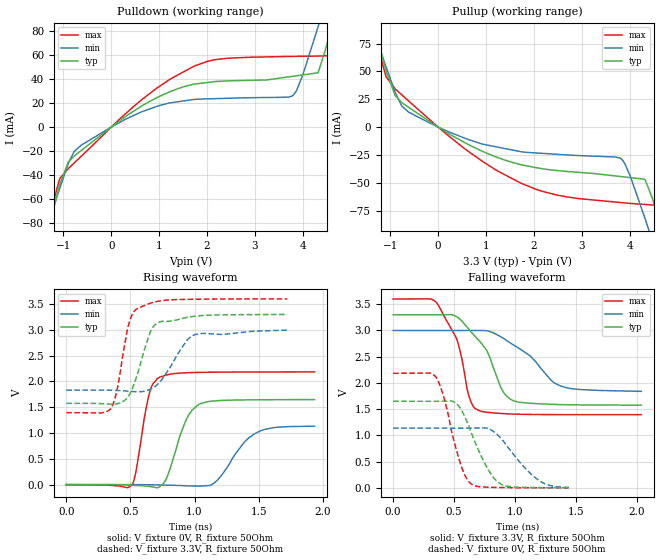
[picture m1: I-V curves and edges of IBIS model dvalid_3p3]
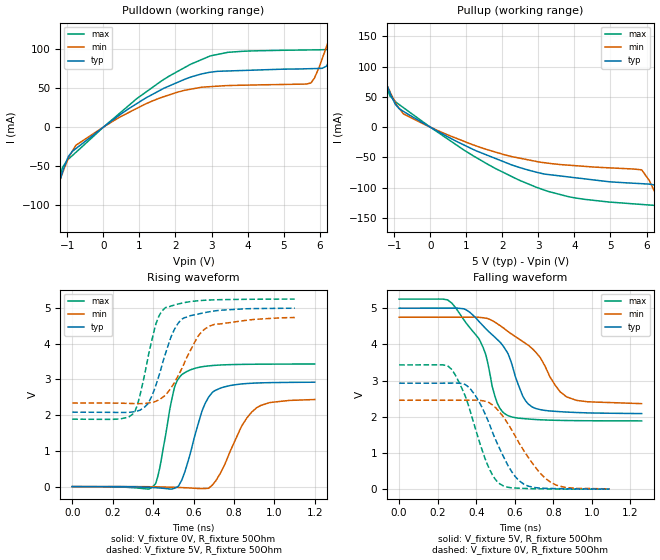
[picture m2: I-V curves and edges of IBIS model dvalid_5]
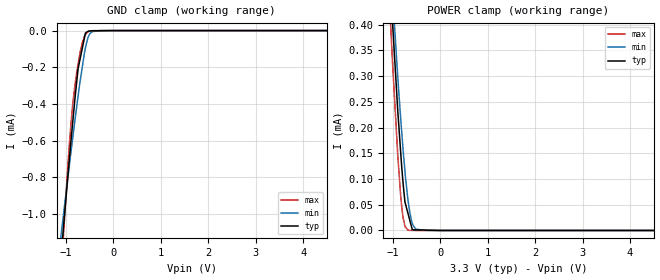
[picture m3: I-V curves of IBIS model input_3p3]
|Texas Instruments Incorporated
| DDC114: Quad Current Input 20-Bit Analog-To-Digital Converter
| Marketing part#   Digital Voltage Range   Package-type   #pins
| DDC114IRTCR   2.7V-5.25V   VQFN   48
| DDC114IRTCRG3   2.7V-5.25V   VQFN   48
| DDC114IRTCT   2.7V-5.25V   VQFN   48
| DDC114IRTCTG3   2.7V-5.25V   VQFN   48
[IBIS Ver]   3.2
[File name]   ddc114.ibs
|SIMDE Ver   V3.0 - 201101 - RHL4 - Build 457
[File Rev]   1.0
[Date]   7/13/2011
[Source]
| Texas Instruments Incorporated.
| Analog-eLab Design Center, HPA
| 12500 TI Blvd
| Dallas, TX -75243
| e-mail: elab_scm_ibis@list.ti.com
[Notes]   Revision History:
| Rev 1.0: 7/13/2011
| - Initial version of the model
| - Model generated from simulations in TISPICE
| - Model matched to SPICE simulation
| - C_comp although listed in numerical order of value are
|   obtained from varying PVT conditions. For PVT conditions for
|   each specific value refer the buffer description under
|   respective [Model]. IBIS model user is responsible for using
|   appropriate C_comp to simulate for Signal Integrity.
| - Model names with a trailing _3p3 contains the model for
|   3.3V [3.0V and 3.6V]. Model names with a trailing _5 contains
|   the model for 5.0V [4.75V and 5.25V].
|*  EXCEPTION:   *
|*  - For model RESET there will be a leakage current in the   *
|*   clamp I-V table because of the pullup on pad.   *
[Disclaimer]
| This model is designed as an aid for customers of Texas Instruments.
| TI and its licensors and suppliers make no warranties, either expressed
| or implied, with respect to this  model, including the warranties of
| merchantability or fitness for a particular purpose. The model is
| provided solely on an "as is" basis. The entire risk as to its quality
| and performance is with the customer.
[Copyright]
 (C) Copyright 2011 Texas Instruments Incorporated.All rights reserved.
|   DDC114
[Component]   DDC114
[Manufacturer]   TI
[Package]   |48 VQFN  -  RTC package
|   typ   min   max
R_pkg   0.07335   0.06625   0.09331
L_pkg   1.25878nH   1.11691nH   1.65971nH
C_pkg   0.40216pF   0.37695pF   0.45725pF
[Pin]  signal_name   model_name   R_pin   L_pin   C_pin
1   DOUT   DOUT_DVALID   0.07718   1.33291nH  0.43988pF
2   _DOUT   DOUT_DVALID   0.07236   1.23651nH  0.40395pF
3   CLK_4X   INPUT   0.06871   1.16431nH  0.40738pF
4   FORMAT   INPUT   0.06661   1.12331nH  0.39420pF
5   HISPD/_LOPWR   INPUT   0.06625   1.11691nH  0.38235pF
6   RANGE0   INPUT   0.06711   1.13471nH  0.37695pF
7   RANGE1   INPUT   0.06859   1.16501nH  0.37885pF
8   RANGE2   INPUT   0.07053   1.20411nH  0.38749pF
9   AGND   GND   0.07256   1.24541nH  0.40171pF
10   VREF   TERM   0.07469   1.28841nH  0.41402pF
11   AGND   GND   0.07881   1.37201nH  0.41890pF
12   AGND   GND   0.09121   1.62491nH  0.46203pF
13   AGND   GND   0.08470   1.49191nH  0.45195pF
14   AGND   GND   0.07477   1.29131nH  0.41332pF
15   AIN4   TERM   0.07121   1.22011nH  0.40949pF
16   AGND   GND   0.07069   1.20981nH  0.40042pF
17   AIN3   TERM   0.06914   1.17901nH  0.38622pF
18   AGND   GND   0.06992   1.19441nH  0.38292pF
19   AGND   GND   0.07038   1.20361nH  0.39011pF
20   AGND   GND   0.07481   1.29231nH  0.39558pF
21   AIN2   TERM   0.07296   1.25531nH  0.40408pF
22   AGND   GND   0.07964   1.38951nH  0.42187pF
23   AIN1   TERM   0.08099   1.41681nH  0.41365pF
24   AGND   GND   0.08669   1.53211nH  0.44910pF
25   AGND   GND   0.08782   1.55561nH  0.45732pF
26   AGND   GND   0.07613   1.31761nH  0.41270pF
27   AVDD   POWER   0.07504   1.29551nH  0.41279pF
28   AGND   GND   0.07369   1.26821nH  0.40112pF
29   DGND   GND   0.07069   1.20751nH  0.38902pF
30   DGND   GND   0.06871   1.16731nH  0.37769pF
31   TEST   INPUT   0.06717   1.13591nH  0.37772pF
32   _RESET   RESET   0.06625   1.11691nH  0.37891pF
33   NC   NC   0.00005   0.00141nH  0.31967pF
34   NC   NC   0.00005   0.00141nH  0.32949pF
35   _DIN   DIN   0.08700   1.53131nH  0.41889pF
36   DIN   DIN   0.09331   1.65971nH  0.45725pF
37   DVDD   POWER   0.08459   1.48251nH  0.44764pF
38   DGND   GND   0.04204   1.02189nH  0.46866pF
39   _DCLK   INPUT   0.08351   1.46051nH  0.42645pF
40   DCLK   INPUT   0.07808   1.35021nH  0.41213pF
41   DGND   GND   0.07472   1.28211nH  0.39060pF
42   CLK   CLK   0.07247   1.23681nH  0.38444pF
43   DGND   GND   0.07058   1.19861nH  0.38161pF
44   _DVALID   DOUT_DVALID   0.06925   1.17211nH  0.38411pF
45   DGND   GND   0.06900   1.16711nH  0.39824pF
46   CONV   INPUT   0.07026   1.19231nH  0.40906pF
47   DGND   GND   0.07318   1.25121nH  0.40470pF
48   DGND   GND   0.07736   1.33561nH  0.43945pF
49   THERMAL_PAD   NC   0.00005   0.00141nH  6.11239pF
[Diff_pin]   inv_pin   vdiff   tdelay_typ   tdelay_min   tdelay_max
1   2   NA   NA   NA   NA
36   35   NA   NA   NA   NA
40   39   NA   NA   NA   NA
|   Model Selectors
[Model Selector] DOUT_DVALID
dvalid_3p3   3.3V digital output
dvalid_5   5.0V digital output
[Model Selector] INPUT
input_3p3   3.3V digital input
input_5   5.0V digital input
[Model Selector] RESET
reset_3p3   3.3V digital input
reset_5   5.0V digital input
[Model Selector] DIN
din_3p3   3.3V digital input
din_5   5.0V digital input
[Model Selector] CLK
clk_3p3   3.3V digital input
clk_5   5.0V digital input
[Model Selector] TERM
term_3-3V   3.3V nominal termination
term_5-0V   5.0V nominal termination
[Model] term_3-3V
Model_type Terminator
C_comp   1.0e-20F  1.0e-20F  1.0e-20F
|   typ   min   max
[Voltage Range]   3.3V   3.0V   3.6V
[POWER Clamp Reference]   3.3V   3.0V   3.6V
[GND Clamp Reference]   0V   0V   0V
|Ambient Temperature   25   85   -40
|Junction Temperature
[Temperature Range]   27   87   -40
[Model] term_5-0V
Model_type Terminator
C_comp   1.0e-20F  1.0e-20F  1.0e-20F
|   typ   min   max
[Voltage Range]   5.0V   4.75V   5.25V
[POWER Clamp Reference]   5.0V   4.75V   5.25V
[GND Clamp Reference]   0V   0V   0V
|Ambient Temperature   25   85   -40
|Junction Temperature
[Temperature Range]   27   87   -40
| Models and submodels in the file (12): dvalid_3p3 (Output), dvalid_5 (Output), input_3p3 (Input), input_5 (Input), reset_3p3 (Input), reset_5 (Input), din_3p3 (Input), din_5 (Input), clk_3p3 (Input), clk_5 (Input), term_3-3V (Terminator), term_5-0V (Terminator)
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|   dvalid_3p3 Model
[Model]   dvalid_3p3
Model_type   Output
Polarity   Non-Inverting
Vmeas = 1.65
Vref = 1.65
Cref = 9pF
Rref = 50
|   typ   min   max
|   (nom PVT)   (fast PVT)   (slow PVT)
|C_comp from frequency sweep method (F=8MHz)
|C_comp   8.990e-13   8.643e-13   9.187e-13
|ON state : BUFFER OUTPUT TURNED HIGH
|C_comp   8.990e-13   8.643e-13   9.187e-13
|OFF state: BUFFER OUTPUT TURNED LOW
|C_comp   8.386e-13   7.914e-13   9.617e-13
|C_comp from LC tank measurement(L=1nH)
|Resonant Frequency(Hz)   9.340e+09   9.530e+09   9.090e+09
C_comp   2.907e-13   2.792e-13   3.069e-13
|ON state : BUFFER OUTPUT TURNED HIGH
|Resonant Frequency(Hz)   9.340e+09   9.530e+09   9.090e+09
|C_comp   2.907e-13   2.792e-13   3.069e-13
|OFF state: BUFFER OUTPUT TURNED LOW
|Resonant Frequency(Hz)   9.920e+09   9.990e+09   9.480e+09
|C_comp   2.577e-13   2.541e-13   2.821e-13
| Where nom  PVT is Nominal Process, 3.3V, 27C
|   Fast PVT is Strong Process,  3.6V, -40C
|   Slow PVT is Weak Process,   3V, 87C
[Voltage Range]   3.3   3   3.6
|Ambient Temperature   25   85   -40
|Junction Temperature
[Temperature Range]   27   87   -40
[Pullup Reference]   3.3   3   3.6
[Pulldown Reference]   0   0   0
[Power Clamp Reference]   3.3   3   3.6
[GND Clamp Reference]   0   0   0
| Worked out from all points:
|   slope of the pulldown table from 0 to 0.495 V, typ, clamps not added: 35.3 ohm
|   slope of the pullup table from 0 to 0.495 V, typ, clamps not added: 39.5 ohm
|   falling waveform, V_fixture 3.3V, R_fixture 50Ohm: 20-80 % time 235ps typ, 331ps min, 167ps max; typ from 3.3 V to 1.58 V
|   rising waveform, V_fixture 0V, R_fixture 50Ohm: 20-80 % time 135ps typ, 199ps min, 89.7ps max; typ from 0 V to 1.65 V
|   rising waveform, V_fixture 3.3V, R_fixture 50Ohm: 20-80 % time 130ps typ, 177ps min, 96.6ps max; typ from 1.58 V to 3.3 V
|   falling waveform, V_fixture 0V, R_fixture 50Ohm: 20-80 % time 190ps typ, 249ps min, 143ps max; typ from 1.65 V to 0.002 V
[Pulldown]
|   Voltage   I(typ)   I(min)   I(max)
-3.3V     -409.1mA   -351.2mA   -450.8mA
-1.409V   -98.56mA   -93.91mA   -95.86mA
-1.307V   -82.51mA   -80.61mA   -77.63mA
-1.069V   -47.29mA   -50.4mA    -42.8mA
-636mV    -19.86mA   -15.41mA   -24.74mA
1.75V     36.04mA    23.17mA    51.28mA
3.78V     42.43mA    26.05mA    59.14mA
4.316V    45.43mA    83.87mA    59.41mA
4.748V    107.6mA    142mA      61.58mA
4.9V      132.2mA    162.7mA    80.33mA
5.168V    175.9mA    199.9mA    128.8mA
6.6V      415mA      398.6mA    399.1mA
[Pullup]
|   Voltage   I(typ)   I(min)   I(max)
-3.3V     414.9mA    356.7mA    456.5mA
-1.435V   104.9mA    99.57mA    103.2mA
-1.087V   50.96mA    53.97mA    45.12mA
-897.6mV  28.24mA    31.11mA    34.26mA
-624mV    17.96mA    13.67mA    23.73mA
1.746V    -34.06mA   -22.28mA   -50.75mA
3.804V    -44.43mA   -27.97mA   -67.79mA
4.316V    -46.91mA   -81.93mA   -69.55mA
4.468V    -63.59mA   -101.9mA   -70mA
4.81V     -115.6mA   -147.6mA   -73.38mA
4.954V    -138.3mA   -167mA     -89.55mA
6.6V      -409.3mA   -392.5mA   -394.1mA
[Ramp]
R_load = 50
|   typ   min   max
dV/dt_r   0.990295/1.3557e-10   0.68271/2.0008e-10   1.31056/8.9629e-11
dV/dt_f   1.0346/2.35346e-10   0.700849/3.32929e-10   1.32291/1.66806e-10
[Falling Waveform]
V_fixture = 3.3V
V_fixture_min = 3V
V_fixture_max = 3.6V
R_fixture = 50Ohm
|   Time   V(typ)   V(min)   V(max)
0s        3.3V       3V         3.6V
358ps     3.3V       3V         3.525V
520ps     3.264V     3V         2.851V
622ps     3.025V     3.001V     1.754V
710ps     2.797V     3V         1.47V
778ps     2.573V     2.991V     1.439V
892ps     1.88V      2.869V     1.417V
986ps     1.664V     2.728V     1.407V
1.37ns    1.588V     1.947V     1.397V
2.038ns   1.577V     1.84V      1.395V
[Rising Waveform]
V_fixture = 0V
V_fixture_min = 0V
V_fixture_max = 0V
R_fixture = 50Ohm
|   Time   V(typ)   V(min)   V(max)
0s        1.108nV    1.352nV    1.021nV
510ps     -11.02mV   559.2uV    -5.106mV
648ps     -35.21mV   -2.127mV   1.774V
726ps     -43.97mV   -6.168mV   2.081V
790ps     174.6mV    -10.63mV   2.13V
940ps     1.285V     -23.37mV   2.168V
1.032ns   1.552V     -27.83mV   2.175V
1.176ns   1.627V     83.58mV    2.179V
1.46ns    1.643V     974.4mV    2.183V
1.934ns   1.648V     1.132V     2.184V
[Rising Waveform]
V_fixture = 3.3V
V_fixture_min = 3V
V_fixture_max = 3.6V
R_fixture = 50Ohm
|   Time   V(typ)   V(min)   V(max)
0s        1.576V     1.831V     1.395V
350ps     1.56V      1.829V     1.477V
398ps     1.568V     1.824V     1.859V
480ps     1.693V     1.811V     3.044V
550ps     2.104V     1.801V     3.406V
654ps     2.954V     1.846V     3.515V
720ps     3.143V     1.964V     3.556V
938ps     3.24V      2.788V     3.59V
996ps     3.262V     2.901V     3.592V
1.722ns   3.297V     2.993V     3.6V
[Falling Waveform]
V_fixture = 0V
V_fixture_min = 0V
V_fixture_max = 0V
R_fixture = 50Ohm
|   Time   V(typ)   V(min)   V(max)
0s        1.651V     1.139V     2.184V
350ps     1.65V      1.139V     2.12V
424ps     1.652V     1.138V     1.666V
520ps     1.603V     1.138V     720mV
582ps     1.39V      1.138V     279.8mV
640ps     1.066V     1.14V      77.63mV
774ps     375.5mV    1.137V     14.08mV
888ps     67.93mV    939.3mV    6.722mV
1.21ns    5.107mV    120.8mV    1.565mV
1.442ns   2.095mV    8.586mV    925.5uV
|   dvalid_5 Model
[Model]   dvalid_5
Model_type   Output
Polarity   Non-Inverting
Vmeas = 2.5
Vref = 2.5
Cref = 9pF
Rref = 50
|   typ   min   max
|   (nom PVT)   (fast PVT)   (slow PVT)
|C_comp from frequency sweep method (F=8MHz)
|C_comp   8.665e-13   7.977e-13   9.259e-13
|ON state : BUFFER OUTPUT TURNED HIGH
|C_comp   8.665e-13   7.977e-13   9.259e-13
|OFF state: BUFFER OUTPUT TURNED LOW
|C_comp   7.892e-13   7.024e-13   8.409e-13
|C_comp from LC tank measurement(L=1nH)
|Resonant Frequency(Hz)   9.120e+09   9.140e+09   9.060e+09
C_comp   3.048e-13   3.035e-13   3.089e-13
|ON state : BUFFER OUTPUT TURNED HIGH
|Resonant Frequency(Hz)   9.120e+09   9.140e+09   9.060e+09
|C_comp   3.048e-13   3.035e-13   3.089e-13
|OFF state: BUFFER OUTPUT TURNED LOW
|Resonant Frequency(Hz)   1.011e+10   1.026e+10   9.970e+09
|C_comp   2.481e-13   2.409e-13   2.551e-13
| Where nom  PVT is Nominal Process, 5V, 27C
|   Fast PVT is Strong Process,  5.25V, -40C
|   Slow PVT is Weak Process,   4.75V, 87C
[Voltage Range]   5   4.75   5.25
|Ambient Temperature   25   85   -40
|Junction Temperature
[Temperature Range]   27   87   -40
[Pullup Reference]   5   4.75   5.25
[Pulldown Reference]   0   0   0
[Power Clamp Reference]   5   4.75   5.25
[GND Clamp Reference]   0   0   0
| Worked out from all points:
|   slope of the pulldown table from 0 to 0.75 V, typ, clamps not added: 29.9 ohm
|   slope of the pullup table from 0 to 0.75 V, typ, clamps not added: 31.1 ohm
|   falling waveform, V_fixture 5V, R_fixture 50Ohm: 20-80 % time 182ps typ, 227ps min, 148ps max; typ from 5 V to 2.09 V
|   rising waveform, V_fixture 0V, R_fixture 50Ohm: 20-80 % time 92.2ps typ, 125ps min, 66.2ps max; typ from 0 V to 2.92 V
|   rising waveform, V_fixture 5V, R_fixture 50Ohm: 20-80 % time 104ps typ, 134ps min, 80.1ps max; typ from 2.08 V to 4.99 V
|   falling waveform, V_fixture 0V, R_fixture 50Ohm: 20-80 % time 150ps typ, 178ps min, 129ps max; typ from 2.93 V to 0.004 V
[Pulldown]
|   Voltage   I(typ)   I(min)   I(max)
-5V       -692.7mA   -587mA     -774.9mA
-2.336V   -249.9mA   -219.4mA   -268.2mA
-1.31V    -83.5mA    -81.13mA   -78.77mA
-1.129V   -56.99mA   -58.26mA   -51.14mA
-760mV    -27.41mA   -23.18mA   -32.26mA
1.149V    36.72mA    29.39mA    44.02mA
2.94V     70.4mA     51.94mA    90.99mA
5.752V    75.1mA     56.65mA    99.19mA
6.195V    78.52mA    104.1mA    99.67mA
6.525V    122.3mA    147.1mA    100.7mA
7.088V    213.8mA    225mA      179.3mA
10V       701.9mA    630.5mA    736.1mA
[Pullup]
|   Voltage   I(typ)   I(min)   I(max)
-5V       701.6mA    595.7mA    784.1mA
-2.336V   253.8mA    223.3mA    272mA
-1.31V    85.41mA    83.11mA    80.69mA
-1.118V   56.75mA    58.47mA    51.53mA
-745.8mV  26.12mA    21.97mA    32.23mA
1.197V    -37.07mA   -29.48mA   -47.61mA
2.94V     -74.48mA   -56.69mA   -99.36mA
5.866V    -93.49mA   -70.89mA   -127.8mA
6.305V    -96.83mA   -117.1mA   -129.6mA
6.82V     -167.4mA   -185mA     -136.9mA
7.103V    -213.4mA   -223.9mA   -181.3mA
10V       -693mA     -621.5mA   -727.7mA
[Ramp]
R_load = 50
|   typ   min   max
dV/dt_r   1.75644/9.25523e-11   1.47285/1.2615e-10   2.05969/6.61752e-11
dV/dt_f   1.75005/1.81489e-10   1.44534/2.28101e-10   2.01827/1.48097e-10
[Falling Waveform]
V_fixture = 5V
V_fixture_min = 4.75V
V_fixture_max = 5.25V
R_fixture = 50Ohm
|   Time   V(typ)   V(min)   V(max)
0s        5V         4.75V      5.25V
274ps     5.001V     4.75V      5.135V
422ps     4.589V     4.744V     4.073V
448ps     4.441V     4.725V     3.74V
509ps     4.135V     4.571V     2.379V
564ps     3.752V     4.359V     2.035V
641ps     2.576V     4.08V      1.953V
692ps     2.267V     3.874V     1.931V
869ps     2.131V     2.55V      1.898V
1.258ns   2.089V     2.364V     1.888V
[Rising Waveform]
V_fixture = 0V
V_fixture_min = 0V
V_fixture_max = 0V
R_fixture = 50Ohm
|   Time   V(typ)   V(min)   V(max)
0s        1.478nV    1.722nV    1.377nV
403ps     -29.3mV    -4.95mV    25.2mV
432ps     -39.61mV   -8.213mV   499.9mV
505ps     -46.91mV   -19.74mV   2.754V
568ps     613.8mV    -34.36mV   3.223V
645ps     2.156V     -53.33mV   3.355V
708ps     2.693V     145.5mV    3.392V
843ps     2.874V     1.736V     3.419V
913ps     2.898V     2.208V     3.423V
1.2ns     2.92V      2.436V     3.43V
[Rising Waveform]
V_fixture = 5V
V_fixture_min = 4.75V
V_fixture_max = 5.25V
R_fixture = 50Ohm
|   Time   V(typ)   V(min)   V(max)
0s        2.082V     2.338V     1.886V
237ps     2.073V     2.333V     1.892V
308ps     2.098V     2.322V     2.08V
334ps     2.136V     2.321V     2.528V
380ps     2.373V     2.341V     3.756V
415ps     2.857V     2.391V     4.568V
465ps     3.786V     2.585V     5.018V
536ps     4.65V      3.231V     5.123V
659ps     4.87V      4.421V     5.213V
1.101ns   4.989V     4.73V      5.246V
[Falling Waveform]
V_fixture = 0V
V_fixture_min = 0V
V_fixture_max = 0V
R_fixture = 50Ohm
|   Time   V(typ)   V(min)   V(max)
0s        2.929V     2.458V     3.433V
270ps     2.93V      2.458V     3.322V
344ps     2.886V     2.458V     2.557V
391ps     2.622V     2.461V     1.756V
462ps     1.881V     2.405V     635.2mV
522ps     1.114V     2.127V     148.7mV
622ps     237.3mV    1.277V     28.24mV
776ps     23.35mV    230mV      8.29mV
873ps     12.47mV    43.53mV    4.725mV
1.092ns   4.272mV    10.34mV    2.297mV
|   input_3p3 Model
[Model]   input_3p3
Model_type   Input
Vinl = 0.66
Vinh = 2.64
|   typ   min   max
|   (nom PVT)   (fast PVT)   (slow PVT)
|C_comp from frequency sweep method (F=19.2MHz)
|Average
|C_comp   5.452e-13   4.673e-13   6.254e-13
|C_comp from LC tank measurement(L=1nH)
|Average
|Resonant Frequency(Hz)   5.974e+10   6.330e+10   4.600e+10
C_comp   7.105e-15   6.328e-15   1.198e-14
| Where nom  PVT is Nominal Process, 3.3V, 27C
|   Fast PVT is Strong Process,  3.6V, -40C
|   Slow PVT is Weak Process,   3V, 87C
[Model Spec]
|Subparameter   typ   min   max
Vinl   0.66   0.60   0.72
Vinh   2.64   2.4   2.88
[Voltage Range]   3.3   3   3.6
|Ambient Temperature   25   85   -40
|Junction Temperature
[Temperature Range]   27   87   -40
[Power Clamp Reference]   3.3   3   3.6
[GND Clamp Reference]   0   0   0
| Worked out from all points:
|   GND clamp passes 1 mA (typ) near -1.03 V on its own axis
|   POWER clamp passes 1 mA (typ) near -1.34 V on its own axis
[GND Clamp]
|   Voltage   I(typ)   I(min)   I(max)
-3.3V     -8.297mA   -6.124mA   -11.81mA
-1.084V   -1.164mA   -1.069mA   -1.242mA
-1.02V    -968.1uA   -929.4uA   -975.6uA
-896.4mV  -604.5uA   -664.1uA   -510.9uA
-810mV    -366.2uA   -484.9uA   -294.7uA
-745.8mV  -208.2uA   -358.1uA   -183.3uA
-658.8mV  -98.99uA   -201.6uA   -69.11uA
-590.7mV  -13.54uA   -94.37uA   -22.97uA
-544.5mV  -5.035uA   -46.28uA   -9.004uA
-447mV    -1.44uA    -5.516uA   -674.8nA
-285mV    -914.5nA   -64.76nA   -169.2nA
6.6V      0A         0A         0A
[POWER Clamp]
|   Voltage   I(typ)   I(min)   I(max)
-3.3V     4.857mA    4.548mA    5.262mA
-1.145V   636.3uA    674.7uA    584.6uA
-1.026V   433.6uA    486.8uA    360.8uA
-1.004V   399.5uA    454.8uA    321.5uA
-897.6mV  233.3uA    299uA      147.3uA
-835.2mV  151.3uA    216.7uA    67.34uA
-788.4mV  95.68uA    160.8uA    26.91uA
-745.8mV  55.41uA    115.4uA    8.775uA
-684mV    33.95uA    60.77uA    842.3nA
-564mV    1.345uA    8.118uA    117.5nA
-285mV    675.8nA    0A         0A
6.6V      0A         0A         0A
